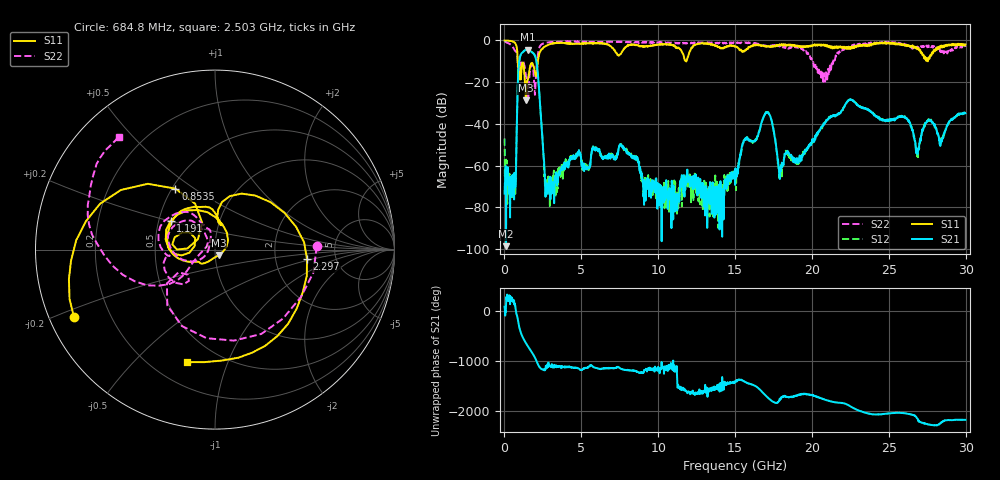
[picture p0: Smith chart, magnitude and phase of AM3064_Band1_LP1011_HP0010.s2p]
# Hz S DB R 50.0
!freq dBS11 angS11 dBS21 angS21 dBS12 angS12 dBS22 angS22
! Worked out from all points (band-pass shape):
!   1600 points, 10 MHz to 29.98 GHz, reference 50 ohm
!   highest |S21| = -4.41 dB at 1.51 GHz (marker M1); lowest = -98.6 dB at 103.7 MHz (marker M2)
!   |S21| within 3 dB of the highest: 1.034 GHz to 1.985 GHz (951.1 MHz wide, 63 % of centre)
!   lowest |S11| = -28.8 dB at 1.397 GHz (marker M3), VSWR 1.08, Z = 51.9 - j3.19 ohm
!   |S11| at or under -10 dB: 865.9 MHz to 2.17 GHz (1.304 GHz wide, 85.9 % of centre); 11.80357 GHz to 11.83105 GHz (27.49 MHz wide, 0.233 % of centre); 27.5249 GHz to 27.53429 GHz (9.393 MHz wide, 0.0341 % of centre)
!   |S22| runs from -28.9 to -0.3 dB; largest |S21 - S12| = 0.0077
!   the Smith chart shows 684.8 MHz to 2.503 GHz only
!   S11 on the Smith chart (normalised r, x): 684.8 MHz: 0.07, -0.23; 853.5 MHz: 0.52, +0.42; 1.191 GHz: 0.58, +0.20; 2.297 GHz: 3.06, -0.45; 2.503 GHz: 0.34, -0.72
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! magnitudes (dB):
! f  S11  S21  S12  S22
! 10 MHz  0.0  -73.4  -47.0  -0.3
! 103.7 MHz  -0.1  -98.6  -57.1  -0.8
! 684.8 MHz  -1.2  -67.8  -67.2  -4.9
! 853.5 MHz  -7.8  -24.6  -24.5  -9.7
! 1.191 GHz  -10.6  -5.7  -5.6  -9.6
! 1.397 GHz  -28.8  -4.5  -4.5  -17.1
! 1.51 GHz  -19.0  -4.4  -4.4  -25.7
! 2.016 GHz  -16.6  -8.1  -8.0  -20.8
! 2.297 GHz  -5.8  -28.6  -28.6  -2.9
! 2.503 GHz  -3.8  -50.7  -50.7  -1.7
! 2.784 GHz  -2.3  -70.8  -67.2  -1.0
! 5.015 GHz  -1.4  -60.1  -57.3  -0.8
! 7.601 GHz  -6.1  -50.3  -49.8  -0.7
! 10 GHz  -2.0  -74.9  -75.1  -1.0
! 15 GHz  -2.8  -69.3  -62.6  -1.4
! 17.05 GHz  -2.9  -34.5  -34.3  -2.9
! 17.95 GHz  -2.3  -60.9  -64.1  -2.4
! 19.99 GHz  -2.8  -48.7  -48.7  -9.4
! 22.48 GHz  -3.6  -28.2  -28.6  -2.7
! 25 GHz  -1.0  -38.6  -37.9  -1.1
! 26.87 GHz  -4.1  -54.6  -52.0  -3.1
! 29.98 GHz  -1.9  -34.9  -34.6  -3.1
